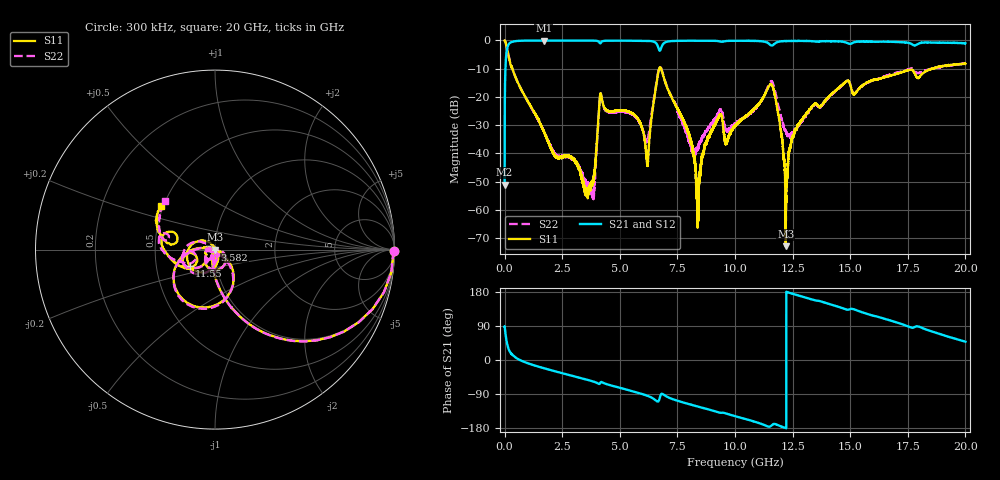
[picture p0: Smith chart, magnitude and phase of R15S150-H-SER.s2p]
!{R15S150}
!Johanson Technology Inc.
!www.johansontechnology.com
!Test Board Conditions:
!Substrate Type  RO4350B
!Substrate Thickness  20 mil
!Substrate Dk  3.66
!TL Type: GCPW
!TL Trace Width  34 mil
!TL Gap  10 mil
!Electrode orientation  Horizontal
!DUT TOPOLOGY	SERIES
!Mounting Pad LxW  26x52 mil
! Created Sat Feb  6 14:12:58 2021
# hz S ma R 50
! 2 Port Network Data from SP1.SP block
! freq  magS11  angS11  magS21  angS21  magS12  angS12  magS22  angS22
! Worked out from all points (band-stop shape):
!   20001 points, 300 kHz to 20 GHz, reference 50 ohm
!   highest |S21| = -0.02 dB at 1.695 GHz (marker M1); lowest = -51.0 dB at 300 kHz (marker M2)
!   |S21| within 3 dB of the highest: 107.3 MHz to 6.692 GHz (6.584 GHz wide, 194 % of centre); 6.781 GHz to end of sweep
!   lowest |S11| = -72.8 dB at 12.2 GHz (marker M3), VSWR 1.00, Z = 50 - j0.0119 ohm
!   |S11| at or under -10 dB: 336.9 MHz to 6.708 GHz (6.371 GHz wide, 181 % of centre); 6.795 GHz to 18.56 GHz (11.77 GHz wide, 92.8 % of centre); 18.56405 GHz to 18.57468 GHz (10.62 MHz wide, 0.0572 % of centre)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
!   |S22| runs from -56.2 to 0.0 dB; largest |S21 - S12| = 0.015
!   S11 on the Smith chart (normalised r, x): 300 kHz: open; 3.582 GHz: 1.00, -0.00; 11.55 GHz: 0.74, -0.14; 20 GHz: 0.49, +0.28
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300000  0.9953 -0.3  0.002817 88.8  0.002801 90.0  0.9947 -0.3
1.033e8  0.7173 -45.4  0.6929 44.5  0.6939 44.3  0.7184 -45.4
1.843e8  0.4984 -62.4  0.8623 27.3  0.8636 27.2  0.4997 -62.4
1.6953e9  0.02477 -126.9  0.9979 -21.5  0.9965 -21.5  0.02544 -93.7
3.3343e9  0.003776 111.9  0.9949 -48.2  0.9952 -48.2  0.004558 -33.8
3.5823e9  0.001958 -178.2  0.9946 -52.2  0.9944 -52.2  0.003021 -82.6
3.8523e9  0.003409 -73.9  0.9924 -56.9  0.9923 -56.9  0.001773 -68.7
4.1873e9  0.1105 -107.3  0.9184 -57.9  0.9186 -58.0  0.1069 -106.7
5.7083e9  0.04502 -173.0  0.9904 -85.0  0.9897 -85.1  0.04291 -168.1
6.1853e9  0.006672 -121.5  0.9832 -94.2  0.9841 -94.2  0.01622 -99.3
6.6673e9  0.269 -75.1  0.757 -109.5  0.7557 -109.4  0.2766 -76.2
7.9363e9  0.02586 158.3  0.9873 -115.3  0.9876 -115.2  0.02113 -172.0
8.3913e9  0.001269 -141.4  0.9899 -122.9  0.9885 -122.8  0.01289 -82.2
9.2803e9  0.04229 -68.8  0.9736 -138.1  0.9744 -138.0  0.05105 -71.0
9.6213e9  0.01514 -84.9  0.9787 -141.3  0.9777 -141.4  0.0256 -95.4
1.00003e10  0.03088 -61.7  0.9866 -148.0  0.9868 -148.1  0.03413 -70.4
1.15453e10  0.1676 -147.7  0.8271 -174.8  0.8279 -174.7  0.1875 -145.2
1.22023e10  0.0002283 -148.5  0.9751 -179.6  0.9764 -179.6  0.02555 171.5
1.25393e10  0.02074 -93.3  0.9789 174.1  0.9807 174.1  0.02198 -137.2
1.33343e10  0.06696 -120.0  0.9717 159.8  0.9718 159.8  0.06573 -120.2
1.66673e10  0.2331 -161.9  0.9505 105.5  0.9385 105.4  0.2436 -168.1
2e10  0.3863 140.8  0.8929 48.3  0.8874 48.0  0.3912 135.7
